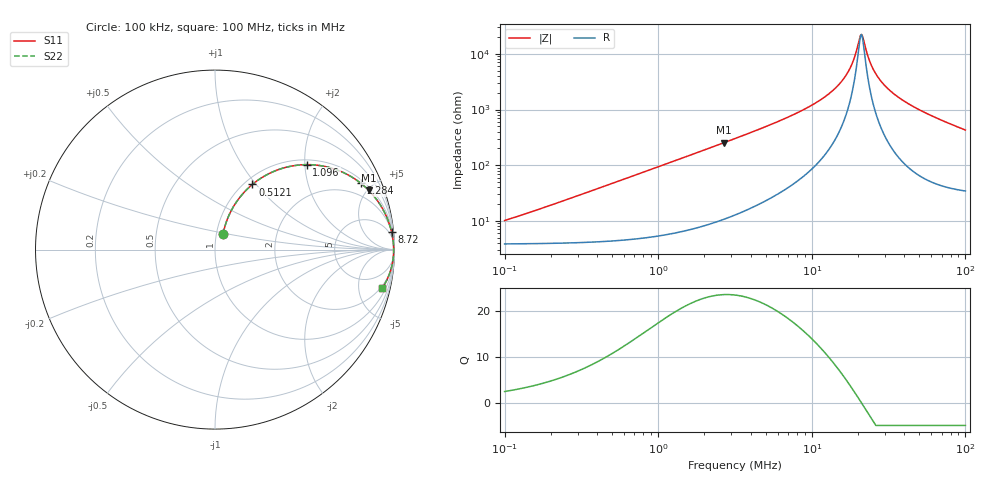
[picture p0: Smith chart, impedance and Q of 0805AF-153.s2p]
# MHz  S  MA  R  50
!Freq  MagS11  AngS11  MagS21  AngS21  MagS12  AngS12  MagS22  AngS22
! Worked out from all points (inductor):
!   801 points, 100 kHz to 100 MHz, reference 50 ohm
!   read as one part in series: L = 14.9 uH near 124.1 kHz
!   highest Q = 23.7 at 2.692 MHz (marker M1), where L = 15 uH
!   self-resonance near 20.87 MHz
!   S11 on the Smith chart (normalised r, x): 100 kHz: 1.08, +0.19; 512.1 kHz: 1.09, +0.96; 1.096 MHz: 1.11, +2.05; 2.284 MHz: 1.18, +4.29; 8.72 MHz: 2, +19; 100 MHz: 1.69, -8.53
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0.1  0.09725 62.5  0.959 -5.2  0.959 -5.2  0.09725 62.5
0.3183882  0.2776 66.2  0.9238 -16.0  0.9238 -16.0  0.2776 66.2
0.5121468  0.4184 60.2  0.871 -24.6  0.871 -24.6  0.4184 60.2
1.004987  0.6662 45.0  0.7088 -41.7  0.7088 -41.7  0.6662 45.0
1.095707  0.697 42.8  0.6802 -44.1  0.6802 -44.1  0.697 42.8
2.284201  0.8922 24.5  0.4151 -63.1  0.4151 -63.1  0.8922 24.5
2.691839  0.9176 21.1  0.3608 -66.5  0.3608 -66.5  0.9176 21.1
3.172224  0.9374 18.1  0.3109 -69.5  0.3109 -69.5  0.9374 18.1
8.719927  0.9885 5.8  0.1015 -80.6  0.1015 -80.6  0.9885 5.8
10.01307  0.9907 4.7  0.08278 -81.2  0.08278 -81.2  0.9907 4.7
13.20312  0.9936 2.8  0.04949 -81.2  0.04949 -81.2  0.9936 2.8
16.10664  0.9949 1.6  0.02798 -78.6  0.02798 -78.6  0.9949 1.6
18.17828  0.9953 0.9  0.01563 -72.0  0.01563 -72.0  0.9953 0.9
20.33982  0.9955 0.2  0.005626 -36.8  0.005626 -36.8  0.9955 0.2
21.05526  0.9955 -0.0  0.004471 1.9  0.004471 1.9  0.9955 -0.0
21.60831  0.9955 -0.2  0.005264 32.0  0.005264 32.0  0.9955 -0.2
23.5589  0.9955 -0.7  0.01249 68.5  0.01249 68.5  0.9955 -0.7
25.2454  0.9954 -1.1  0.01935 75.7  0.01935 75.7  0.9954 -1.1
28.0042  0.9951 -1.7  0.03008 79.7  0.03008 79.7  0.9951 -1.7
31.88044  0.9944 -2.5  0.04406 81.4  0.04406 81.4  0.9944 -2.5
49.53911  0.9887 -5.6  0.09841 80.6  0.09841 80.6  0.9887 -5.6
100  0.9569 -12.9  0.2236 72.5  0.2236 72.5  0.9569 -12.9
